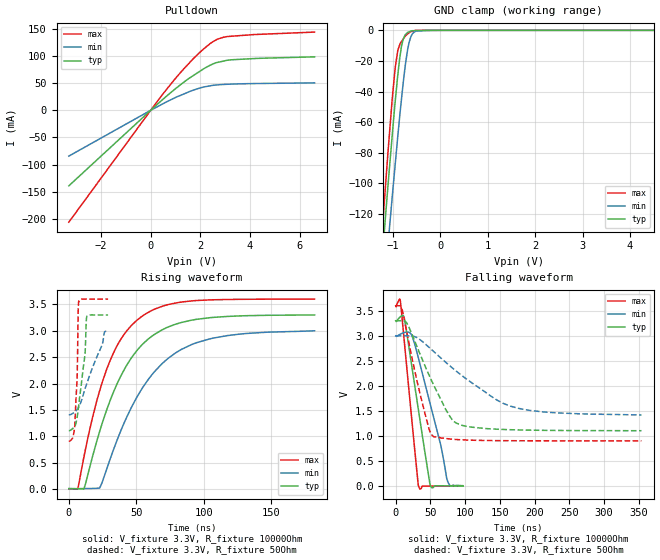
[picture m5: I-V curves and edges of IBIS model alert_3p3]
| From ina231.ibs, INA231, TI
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|   alert_3p3 Model
[Model]   alert_3p3
Model_type   Open_drain
Polarity   Non-Inverting
Vmeas = 1.65
Vref = 3.3
Cref = 2pF
Rref = 10000
|   typ   min   max
|   (nom PVT)   (fast PVT)   (slow PVT)
|C_comp from frequency sweep method (F=50KHz)
|C_comp   2.725e-10   2.376e-10   3.026e-10
|ON state : BUFFER OUTPUT TURNED LOW
|C_comp   2.725e-10   2.376e-10   3.026e-10
|OFF state: BUFFER IN HIGH IMPEDANCE
|C_comp   2.405e-12   2.012e-12   2.826e-12
|C_comp from LC tank measurement(L=1nH)
|Resonant Frequency(Hz)   5.580e+09   5.710e+09   5.200e+09
C_comp   8.143e-13   7.777e-13   9.377e-13
|ON state : BUFFER OUTPUT TURNED LOW
|Resonant Frequency(Hz)   5.580e+09   5.710e+09   5.200e+09
|C_comp   8.143e-13   7.777e-13   9.377e-13
|OFF state: BUFFER IN HIGH IMPEDANCE
|Resonant Frequency(Hz)   4.900e+09   5.620e+09   4.490e+09
|C_comp   1.056e-12   8.028e-13   1.258e-12
| Where nom  PVT is Nominal Process, 3.3V, 27C
|   Fast PVT is Strong Process,  3.6V, -40C
|   Slow PVT is Weak Process,   3V, 125C
[Voltage Range]   3.3   3   3.6
|Ambient Temperature   25   150   -65
|Junction Temperature
[Temperature Range]   27   125   -40
[Pullup Reference]   3.3   3   3.6
[Pulldown Reference]   0   0   0
[Power Clamp Reference]   3.3   3   3.6
[GND Clamp Reference]   0   0   0
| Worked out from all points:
|   slope of the pulldown table from 0 to 0.495 V, typ, clamps not added: 24.4 ohm
|   GND clamp passes 1 mA (typ) near -0.66 V on its own axis
|   falling waveform, V_fixture 3.3V, R_fixture 10000Ohm: 20-80 % time 21.7ns typ, 32.3ns min, 15ns max; typ from 3.3 V to 0.008 V
|   rising waveform, V_fixture 3.3V, R_fixture 10000Ohm: 20-80 % time 32.9ns typ, 39ns min, 27.5ns max; typ from 0.008 V to 3.3 V
|   falling waveform, V_fixture 3.3V, R_fixture 50Ohm: 20-80 % time 43.1ns typ, 88.8ns min, 26.2ns max; typ from 3.3 V to 1.11 V
|   rising waveform, V_fixture 3.3V, R_fixture 50Ohm: 20-80 % time 5.35ns typ, 13.8ns min, 1.91ns max; typ from 1.11 V to 3.3 V
[Pulldown]
|   Voltage   I(typ)   I(min)   I(max)
-3.3V     -139.2mA   -84.44mA   -206.2mA
18mV      754.8uA    460uA      1.129mA
633.6mV   25.87mA    15.47mA    38.31mA
1.246V    48.71mA    28.37mA    71.97mA
1.706V    63.73mA    36.9mA     94.61mA
2.383V    82.71mA    45.01mA    122.4mA
2.678V    88.09mA    46.7mA     130.9mA
3.089V    92.24mA    47.94mA    135.9mA
4.316V    95.63mA    49.31mA    139.8mA
6.6V      98.43mA    50.48mA    144mA
[GND Clamp]
|   Voltage   I(typ)   I(min)   I(max)
-3.3V     -994.3mA   -972.8mA   -1.055A
-1.231V   -151.3mA   -186.9mA   -133.5mA
-1.155V   -121.2mA   -158.8mA   -101.3mA
-1.086V   -94.78mA   -134mA     -72.68mA
-1.015V   -69.11mA   -109.2mA   -45.22mA
-950.4mV  -46.18mA   -87.25mA   -24.23mA
-896.4mV  -29.11mA   -69.03mA   -13.05mA
-818.4mV  -10.43mA   -44.77mA   -7.302mA
-683.1mV  -1.259mA   -11.64mA   -2.218mA
-579mV    -257.7uA   -1.875mA   -510.3uA
-285mV    -126.1uA   -986.3nA   -2.437uA
6.6V      0A         0A         0A
[POWER Clamp]
|   Voltage   I(typ)   I(min)   I(max)
-3.3V     0A         0A         0A
0V        0A         0A         0A
6.6V      0A         0A         0A
[Ramp]
R_load = 10000
|   typ   min   max
dV/dt_r   1.97533/3.28714e-08   1.79298/3.89804e-08   2.15656/2.7487e-08
dV/dt_f   1.97533/2.17263e-08   1.79297/3.23135e-08   2.15656/1.50171e-08
[Falling Waveform]
V_fixture = 3.3V
V_fixture_min = 3V
V_fixture_max = 3.6V
R_fixture = 10000Ohm
|   Time   V(typ)   V(min)   V(max)
0s        3.3V       3V         3.6V
6.9ns     3.382V     3.035V     3.676V
12.7ns    3.334V     3.068V     2.844V
22.85ns   2.428V     3.018V     1.377V
32.5ns    1.546V     2.569V     24.63mV
33.8ns    1.428V     2.499V     -30.74mV
50.85ns   -8.229mV   1.579V     6.694mV
64.65ns   10.36mV    837mV      6.252mV
74.9ns    9.451mV    98.22mV    6.094mV
97.03ns   7.947mV    13.01mV    5.749mV
[Rising Waveform]
V_fixture = 3.3V
V_fixture_min = 3V
V_fixture_max = 3.6V
R_fixture = 10000Ohm
|   Time   V(typ)   V(min)   V(max)
0s        7.784mV    11.69mV    5.725mV
6.5ns     5.853mV    10.49mV    0V
11.2ns    6.756mV    11.28mV    610.5mV
22.85ns   1.094V     20.75mV    1.863V
36.85ns   2.055V     999.8mV    2.768V
53.45ns   2.714V     1.873V     3.261V
71.9ns    3.053V     2.442V     3.485V
94.8ns    3.218V     2.776V     3.574V
126.7ns   3.282V     2.938V     3.596V
182.1ns   3.3V       3V         3.6V
[Falling Waveform]
V_fixture = 3.3V
V_fixture_min = 3V
V_fixture_max = 3.6V
R_fixture = 50Ohm
|   Time   V(typ)   V(min)   V(max)
0s        3.3V       3V         3.6V
8.8ns     3.301V     3.001V     3.55V
18.35ns   3.194V     3V         2.906V
37.25ns   2.563V     2.9V       1.723V
48.7ns    2.197V     2.763V     1.111V
55.3ns    2.002V     2.68V      986.6mV
81.2ns    1.331V     2.365V     940.3mV
95.65ns   1.215V     2.205V     927mV
177ns     1.125V     1.554V     909mV
353.9ns   1.109V     1.423V     907.5mV
[Rising Waveform]
V_fixture = 3.3V
V_fixture_min = 3V
V_fixture_max = 3.6V
R_fixture = 50Ohm
|   Time   V(typ)   V(min)   V(max)
0s        1.109V     1.41V      907.8mV
2.9ns     1.149V     1.435V     974.8mV
4.35ns    1.193V     1.461V     1.177V
6.15ns    1.362V     1.509V     2.107V
6.95ns    1.506V     1.54V      3.362V
7.35ns    1.592V     1.557V     3.557V
12.05ns   2.575V     1.905V     3.6V
13.2ns    3.259V     1.991V     3.6V
26.45ns   3.3V       2.976V     3.6V
29.1ns    3.3V       3V         3.6V
